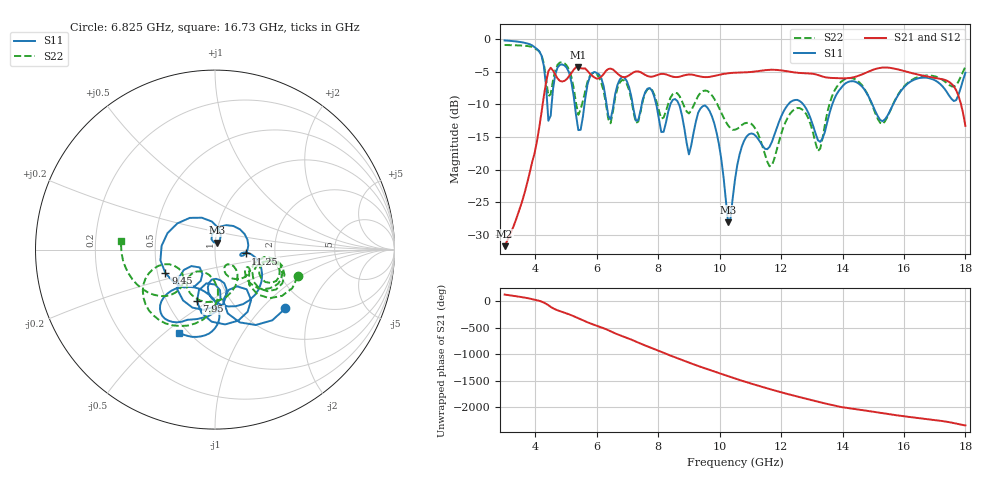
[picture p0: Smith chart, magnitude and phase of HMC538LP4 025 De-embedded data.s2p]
! Chelmsford, MA 01824
! http://www.hittite.com
! Tel: 978-250-3343
! Fax: 978-250-3373
! Device  :  HMC538LP4
! Description:  600 Analog Phase Shifter
! Frequency  :  6.0 GHz - 15.0 GHz
! Package  :  LP4  - 4x4 mm Quad Flatpack No-Lead (QFN) Plastic Package: 24 pin
! Ports  :  2 RF, 1 DC
!  Pin  3  = Rfin  = Port 1
!  Pin  16  = Rfout = Port 2
!  pin  21  = vCTL
! Voltages:  VCTL  = 0 to 5.0 Volts
! Currents :  Vb(V)  Vd(V)  Ib(mA)  Id(mA)
!  0.00  2.50  0.000000	0.471880
! Data:  The device was measured on evaluation board 111296-1.
!  Data was collected using a calibrated network analyzer.
!  The evaluation circuit board was modeled and simulated.This was use
!  to removed the evaluation board circuit from the measured data.
!  The reference plane is the center of the package pin.
! Misc:  Lot #
!Date Measured:  03 - 11 -2009
! Date:  03 - 17 -2009
! Note:
!  Hittite Microwave supplies this data as a sample of measured data at the
!  package pin for this package product.  Your particular data for this product
!  may vary.
!  Data was taken at 25 degrees C.
!  Hittite Microwave reserves the right to change this data at anytime.
# MHz S MA R 50
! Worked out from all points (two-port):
!   201 points, 3 GHz to 18 GHz, reference 50 ohm
!   highest |S21| = -4.31 dB at 5.4 GHz (marker M1); lowest = -31.7 dB at 3 GHz (marker M2)
!   |S21| within 3 dB of the highest: 4.326 GHz to 17.63 GHz (13.3 GHz wide, 121 % of centre)
!   lowest |S11| = -28.1 dB at 10.28 GHz (marker M3), VSWR 1.08, Z = 50.8 + j3.91 ohm
!   |S11| at or under -10 dB: 8.673 GHz to 12.24 GHz (3.563 GHz wide, 34.1 % of centre); 12.72 GHz to 13.67 GHz (948.6 MHz wide, 7.19 % of centre); 14.97 GHz to 15.65 GHz (681.4 MHz wide, 4.45 % of centre)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
!   |S22| runs from -19.5 to -0.9 dB; largest |S21 - S12| = 0.0015
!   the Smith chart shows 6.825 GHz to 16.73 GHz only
!   S11 on the Smith chart (normalised r, x): 6.825 GHz: 1.55, -1.37; 7.95 GHz: 0.70, -0.45; 9.45 GHz: 0.55, -0.16; 11.25 GHz: 1.41, -0.06; 16.73 GHz: 0.45, -0.56
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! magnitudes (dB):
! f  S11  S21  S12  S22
! 3 GHz  -0.2  -31.7  -31.7  -0.9
! 4.125 GHz  -1.9  -13.6  -13.6  -1.9
! 4.425 GHz  -12.5  -4.9  -4.9  -8.8
! 4.875 GHz  -3.9  -6.5  -6.5  -3.6
! 5.4 GHz  -14.0  -4.3  -4.3  -11.6
! 5.55 GHz  -11.9  -4.5  -4.5  -9.4
! 5.925 GHz  -5.1  -5.9  -5.9  -5.2
! 6.45 GHz  -12.3  -4.5  -4.5  -12.9
! 6.825 GHz  -5.8  -5.8  -5.8  -6.3
! 7.95 GHz  -10.3  -5.6  -5.6  -9.7
! 8.025 GHz  -12.3  -5.4  -5.4  -11.0
! 8.625 GHz  -9.5  -5.8  -5.8  -8.3
! 9 GHz  -17.7  -5.4  -5.4  -11.4
! 9.45 GHz  -10.3  -5.8  -5.8  -8.0
! 10.28 GHz  -28.1  -5.3  -5.3  -13.2
! 10.5 GHz  -21.5  -5.2  -5.2  -13.9
! 11.25 GHz  -15.3  -4.9  -4.9  -14.5
! 13.05 GHz  -13.4  -5.4  -5.4  -14.5
! 14.1 GHz  -6.8  -6.0  -6.0  -6.1
! 15.53 GHz  -11.2  -4.4  -4.4  -11.3
! 16.73 GHz  -5.9  -5.7  -5.7  -5.6
! 18 GHz  -5.2  -13.3  -13.3  -4.2
